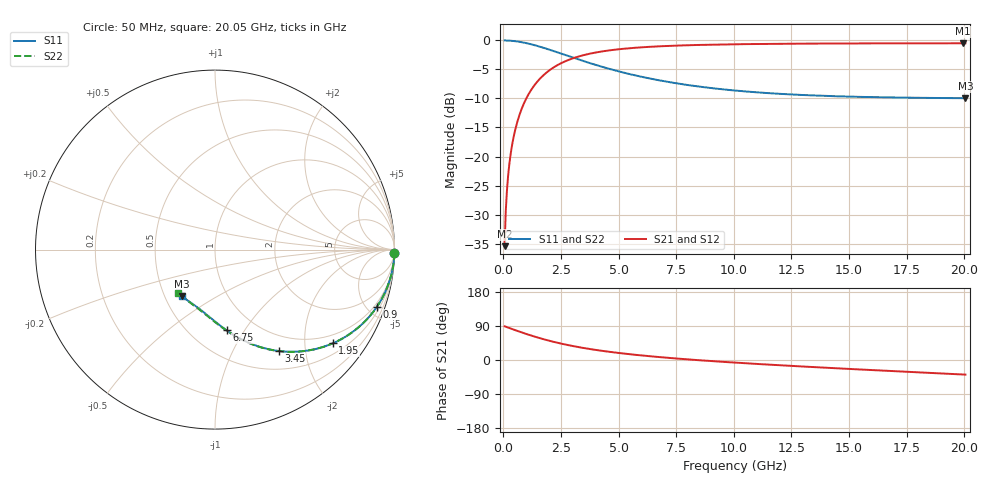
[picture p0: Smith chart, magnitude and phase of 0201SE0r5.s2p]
! AVX Thin Film Operation		Date: August 2001
! Description: Accu-P® Series, Thin Film, SMD, RF Capacitor
! Part Number: 02013J0R5ABW
! 50 MHz  -  20.05 GHz
! Serial Measurements
# mhz S db R 50
!	S11		S21		S12		S22
!	dB	Phase	dB	Phase	dB	Phase	dB	Phase
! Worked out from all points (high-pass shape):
!   401 points, 50 MHz to 20.05 GHz, reference 50 ohm
!   highest |S21| = -0.49 dB at 19.95 GHz (marker M1); lowest = -35.5 dB at 50 MHz (marker M2)
!   |S21| within 3 dB of the highest: 2.741 GHz to end of sweep
!   lowest |S11| = -10.0 dB at 20.05 GHz (marker M3), VSWR 1.93, Z = 30.5 - j17.5 ohm
!   |S11| at or under -10 dB: nowhere
!   |S22| runs from -10.0 to 0.0 dB; largest |S21 - S12| = 0
!   S11 on the Smith chart (normalised r, x): 50 MHz: open; 900 MHz: 0.76, -5.75; 1.95 GHz: 0.76, -2.67; 3.45 GHz: 0.76, -1.53; 6.75 GHz: 0.74, -0.83; 20.05 GHz: 0.61, -0.35
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50  -0.00 -1.1  -35.45 88.9  -35.45 88.9  -0.00 -1.1
100  -0.01 -2.2  -29.43 87.8  -29.43 87.8  -0.01 -2.2
200  -0.02 -4.4  -23.43 85.6  -23.43 85.6  -0.02 -4.4
250  -0.03 -5.5  -21.50 84.5  -21.50 84.5  -0.03 -5.5
350  -0.06 -7.7  -18.61 82.3  -18.61 82.3  -0.06 -7.7
450  -0.10 -9.9  -16.47 80.1  -16.47 80.1  -0.10 -9.9
600  -0.17 -13.1  -14.05 76.8  -14.05 76.8  -0.17 -13.1
900  -0.38 -19.4  -10.75 70.6  -10.75 70.6  -0.38 -19.4
1350  -0.81 -28.2  -7.69 61.8  -7.69 61.8  -0.81 -28.2
1950  -1.53 -38.5  -5.28 51.4  -5.28 51.4  -1.53 -38.6
2600  -2.40 -48.0  -3.73 42.0  -3.73 42.0  -2.40 -48.0
3400  -3.46 -57.4  -2.61 32.5  -2.61 32.5  -3.46 -57.5
3450  -3.52 -57.9  -2.56 32.0  -2.56 32.0  -3.52 -58.0
4150  -4.39 -64.6  -1.98 25.3  -1.98 25.3  -4.39 -64.7
4900  -5.22 -70.5  -1.56 19.3  -1.56 19.3  -5.22 -70.7
6750  -6.86 -81.9  -1.01 7.8  -1.01 7.8  -6.87 -82.3
8300  -7.85 -89.2  -0.79 0.3  -0.79 0.3  -7.86 -89.8
10050  -8.63 -96.1  -0.66 -6.9  -0.66 -6.9  -8.64 -97.2
13400  -9.47 -107.1  -0.54 -18.5  -0.54 -18.5  -9.49 -109.2
16750  -9.82 -116.8  -0.50 -28.9  -0.50 -28.9  -9.85 -120.2
19950  -9.95 -125.5  -0.49 -38.3  -0.49 -38.3  -9.99 -130.1
20050  -9.95 -125.7  -0.49 -38.6  -0.49 -38.6  -9.99 -130.4
